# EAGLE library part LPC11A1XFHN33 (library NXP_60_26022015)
32-bit ARM Cortex-M0 microcontroller; up to 32 kB flash, 8 kB SRAM, 4 kB EEPROM; configurable analog/mixed-signal The LPC11Axx are an ARM Cortex-M0 based, low-cost 32-bit MCU family, designed for 8/16-bit microcontroller applications, offering performance, low power, simple instruction set and memory addressing together with reduced code size compared to existing 8/16-bit architectures. The LPC11Axx operate at CPU frequencies of up to 50 MHz. Analog/mixed-signal subsystems can be configured by software from interconnected digital and analog peripherals. The digital peripherals on the LPC11Axx include up to 32 kB of flash memory, up to 4 kB of EEPROM data memory, up to 8 kB of SRAM data memory, a Fast-mode Plus I 2 C-bus interface, a RS-485/EIA-485 USART, two SSP controllers, four general purpose counter/timers, and up to 42 general purpose I/O pins. Analog peripherals include a 10-bit ADC, a 10-bit DAC, an analog comparator, a temperature sensor, an internal voltage reference, and UnderVoltage LockOut (UVLO) protection. AAL Eindhoven MK
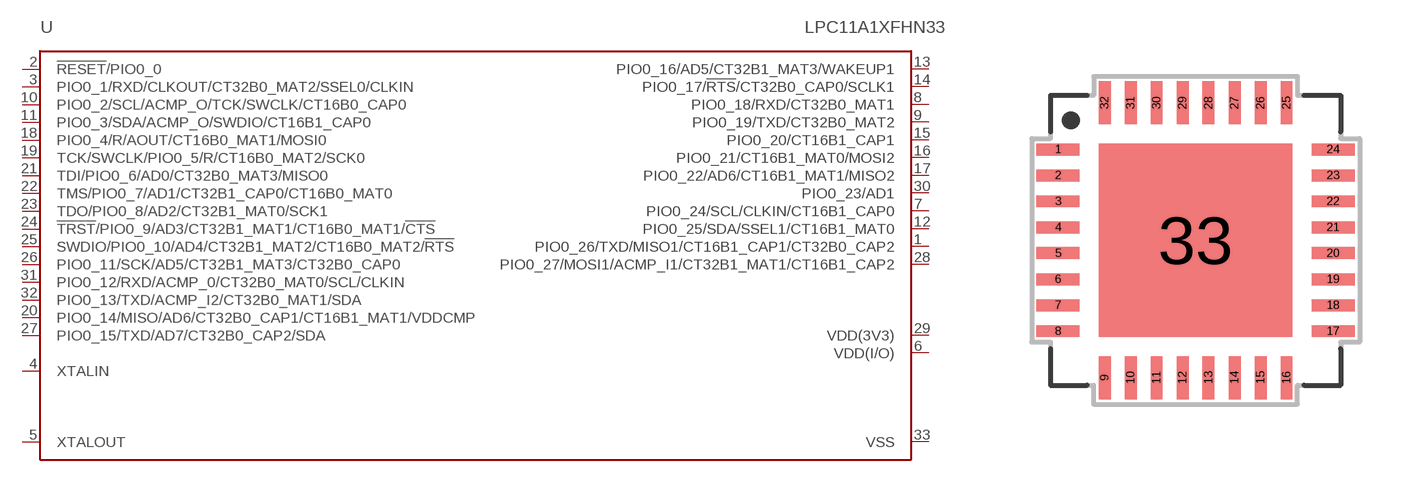
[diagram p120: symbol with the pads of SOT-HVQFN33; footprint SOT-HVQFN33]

Designator prefix U

## LPC11A1XFHN33  [SOT-HVQFN33]
1  PIO0_26/TXD/MISO1/CT16B1_CAP1/CT32B0_CAP2
2  !RESET!/PIO0_0
3  PIO0_1/RXD/CLKOUT/CT32B0_MAT2/SSEL0/CLKIN
4  XTALIN  pas
5  XTALOUT  pas
6  VDD(I/O)  pwr
7  PIO0_24/SCL/CLKIN/CT16B1_CAP0
8  PIO0_18/RXD/CT32B0_MAT1
9  PIO0_19/TXD/CT32B0_MAT2
10  PIO0_2/SCL/ACMP_O/TCK/SWCLK/CT16B0_CAP0
11  PIO0_3/SDA/ACMP_O/SWDIO/CT16B1_CAP0
12  PIO0_25/SDA/SSEL1/CT16B1_MAT0
13  PIO0_16/AD5/CT32B1_MAT3/WAKEUP1
14  PIO0_17/!RTS!/CT32B0_CAP0/SCLK1
15  PIO0_20/CT16B1_CAP1
16  PIO0_21/CT16B1_MAT0/MOSI2
17  PIO0_22/AD6/CT16B1_MAT1/MISO2
18  PIO0_4/R/AOUT/CT16B0_MAT1/MOSI0
19  TCK/SWCLK/PIO0_5/R/CT16B0_MAT2/SCK0
20  PIO0_14/MISO/AD6/CT32B0_CAP1/CT16B1_MAT1/VDDCMP
21  TDI/PIO0_6/AD0/CT32B0_MAT3/MISO0
22  TMS/PIO0_7/AD1/CT32B1_CAP0/CT16B0_MAT0
23  TDO/PIO0_8/AD2/CT32B1_MAT0/SCK1
24  !TRST!/PIO0_9/AD3/CT32B1_MAT1/CT16B0_MAT1/!CTS!
25  SWDIO/PIO0_10/AD4/CT32B1_MAT2/CT16B0_MAT2/!RTS!
26  PIO0_11/SCK/AD5/CT32B1_MAT3/CT32B0_CAP0
27  PIO0_15/TXD/AD7/CT32B0_CAP2/SDA
28  PIO0_27/MOSI1/ACMP_I1/CT32B1_MAT1/CT16B1_CAP2
29  VDD(3V3)  pwr
30  PIO0_23/AD1
31  PIO0_12/RXD/ACMP_0/CT32B0_MAT0/SCL/CLKIN
32  PIO0_13/TXD/ACMP_I2/CT32B0_MAT1/SDA
33  VSS  pwr

## Footprint SOT-HVQFN33 (pad centres in mm)
SOTxxx HVQFN33: plastic thermal enhanced very thin quad flat package; no leads; 33 terminals; body 7 x 7 x 0.85 mm JEDEC: --- IEC: --- Package according LPC111x datasheet
smd 1.075 x 0.3: 1 -3.438,2.275; 2 -3.438,1.625; 3 -3.438,0.975; 4 -3.438,0.325; 5 -3.438,-0.325; 6 -3.438,-0.975; 7 -3.438,-1.625; 8 -3.438,-2.275; 17 3.438,-2.275; 18 3.438,-1.625; 19 3.438,-0.975; 20 3.438,-0.325; 21 3.438,0.325; 22 3.438,0.975; 23 3.438,1.625; 24 3.438,2.275
smd 0.3 x 1.075: 9 -2.275,-3.438; 10 -1.625,-3.438; 11 -0.975,-3.438; 12 -0.325,-3.438; 13 0.325,-3.438; 14 0.975,-3.438; 15 1.625,-3.438; 16 2.275,-3.438; 25 2.275,3.438; 26 1.625,3.438; 27 0.975,3.438; 28 0.325,3.438; 29 -0.325,3.438; 30 -0.975,3.438; 31 -1.625,3.438; 32 -2.275,3.438
smd 4.85 x 4.85: 33 0,0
